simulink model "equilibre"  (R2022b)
settings: Solver=VariableStepAuto  StartTime=0.0  StopTime=10.0  RelTol=1e-3

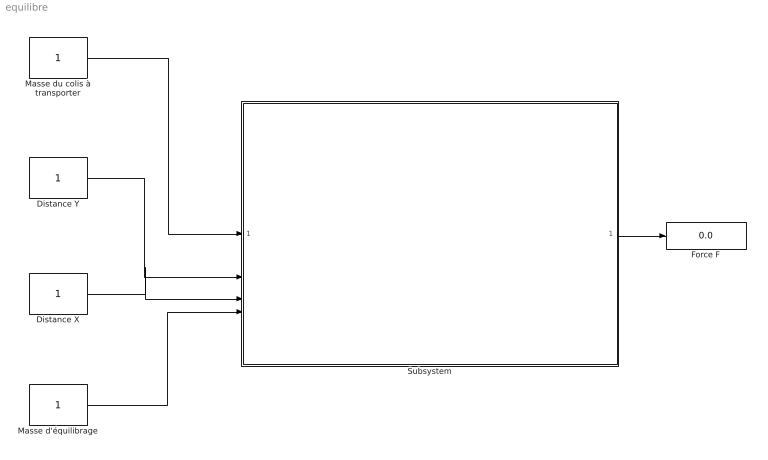
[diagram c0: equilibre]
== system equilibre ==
  Distance X : Constant
  Distance Y : Constant
  Force F : Display
  Masse d'équilibrage : Constant
  Masse du colis à transporter : Constant
  Subsystem : Subsystem
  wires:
  Masse du colis à transporter/1 -> Subsystem/1(In1)
  Distance Y/1 -> Subsystem/2(In2)
  Distance X/1 -> Subsystem/3(In3)
  Masse d'équilibrage/1 -> Subsystem/4(In4)
  Subsystem/1(Out2) -> Force F/1

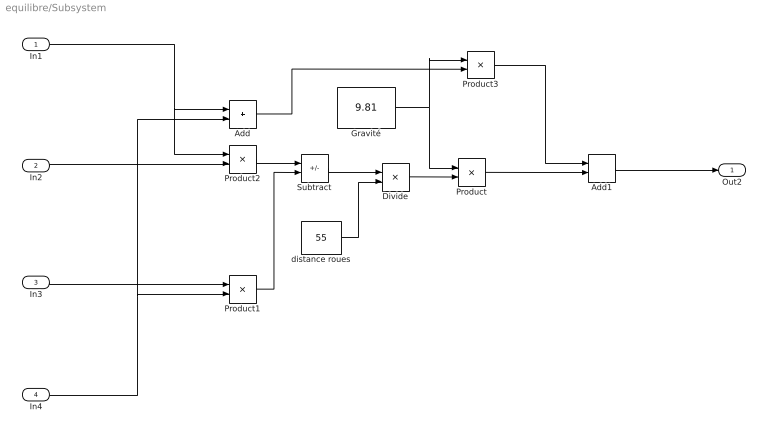
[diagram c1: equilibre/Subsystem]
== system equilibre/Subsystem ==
  In1 : Inport
  In2 : Inport  Port=2
  In3 : Inport  Port=3
  In4 : Inport  Port=4
  Add : Sum
  Add1 : Sum
  Divide : Product  Inputs=*/
  Gravité : Constant  Value=9.81
  Product{,1..3} (4 alike) : Product
  Subtract : Sum  Inputs=+-
  distance roues : Constant  Value=55
  Out2 : Outport
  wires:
  Product2/1 -> Subtract/1
  Subtract/1 -> Divide/1
  Product1/1 -> Subtract/2
  Divide/1 -> Product/2
  distance roues/1 -> Divide/2
  In4/1 -> Product1/2, Add/2
  In1/1 -> Product2/1, Add/1
  Gravité/1 -> Product3/1, Product/1
  In2/1 -> Product2/2
  In3/1 -> Product1/1
  Add/1 -> Product3/2
  Product3/1 -> Add1/1
  Product/1 -> Add1/2
  Add1/1 -> Out2/1
